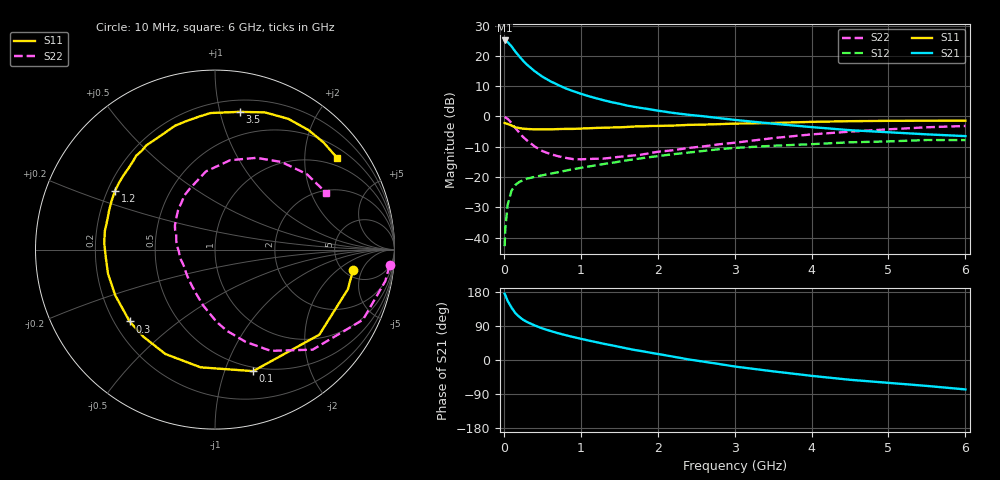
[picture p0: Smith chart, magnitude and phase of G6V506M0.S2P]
! SIEMENS Small Signal Semiconductors
! BFG193
! Si NPN RF Bipolar Junction Transistor in SOT223
! VCE = 0.5 V  IC = 6 mA
! Common Emitter S-Parameters:  August  1996
# GHz  S  MA  R  50
!  f  S11  S21  S12  S22
! GHz  MAG  ANG  MAG  ANG  MAG  ANG  MAG  ANG
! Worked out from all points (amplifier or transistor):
!   36 points, 10 MHz to 6 GHz, reference 50 ohm
!   highest |S21| = 25.1 dB at 10 MHz (marker M1)
!   |S21| within 3 dB of that: start of sweep to 129.9 MHz
!   unconditionally stable (mu >= 1): 941.7 MHz to 4.396 GHz; 5.149 GHz to end of sweep
!   at 250 MHz: K = 0.41, MSG = 19.7 dB, |S12| = -21.1 dB
!   at 1.4 GHz: K = 1.12, MAG = 8.0 dB, |S12| = -15.3 dB
!   at 6 GHz: K = 1.01, MAG = 0.1 dB, |S12| = -7.8 dB
!   S11 on the Smith chart (normalised r, x): 10 MHz: 6.02, -3.42; 100 MHz: 0.46, -1.25; 300 MHz: 0.26, -0.34; 1.2 GHz: 0.23, +0.26; 3.5 GHz: 0.29, +1.15; 6 GHz: 0.76, +2.82
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0.01  0.7778 -8.3  17.98 174.8  0.0072 88.1  0.977 -5.2
0.02  0.7725 -16.6  17.81 170.8  0.0147 83.2  0.9648 -10.5
0.05  0.7501 -39.2  16.82 155.7  0.0348 70.0  0.9123 -25.4
0.1  0.7096 -72.6  14.38 138.3  0.0595 56.3  0.7789 -45.7
0.15  0.6608 -97.0  11.73 123.7  0.0739 46.4  0.6436 -61.2
0.2  0.644 -115.4  9.863 114.1  0.0826 41.0  0.5409 -71.7
0.25  0.6284 -129.4  8.332 106.3  0.0885 37.3  0.4575 -81.6
0.3  0.6216 -139.9  7.177 100.4  0.0937 35.0  0.4024 -88.8
0.4  0.6114 -155.4  5.6 91.3  0.1004 32.8  0.3195 -101.7
0.5  0.6112 -167.2  4.548 83.4  0.1067 31.7  0.2686 -112.7
0.6  0.6099 -175.8  3.844 77.0  0.1131 31.8  0.2398 -122.3
0.8  0.6224 170.4  2.918 65.7  0.1269 31.5  0.2072 -140.7
0.9  0.6224 164.5  2.617 60.7  0.1343 31.4  0.1974 -148.8
1.1  0.6375 154.3  2.164 51.5  0.1487 31.1  0.1983 -163.5
1.2  0.6463 149.5  1.996 47.2  0.1564 30.8  0.2 -170.4
1.6  0.6702 133.2  1.513 30.5  0.1882 26.7  0.2211 167.2
2.2  0.7063 114.0  1.144 8.9  0.2375 17.7  0.2766 141.5
2.8  0.7461 96.9  0.938 -10.6  0.2877 6.4  0.3469 119.4
3.5  0.7795 79.9  0.759 -29.9  0.3282 -9.5  0.4386 96.6
4.5  0.8353 60.7  0.593 -52.2  0.374 -27.9  0.5609 65.7
5.5  0.8499 44.5  0.506 -68.4  0.4081 -49.8  0.6623 39.4
6  0.8507 36.8  0.473 -77.6  0.4071 -62.4  0.6963 26.9
